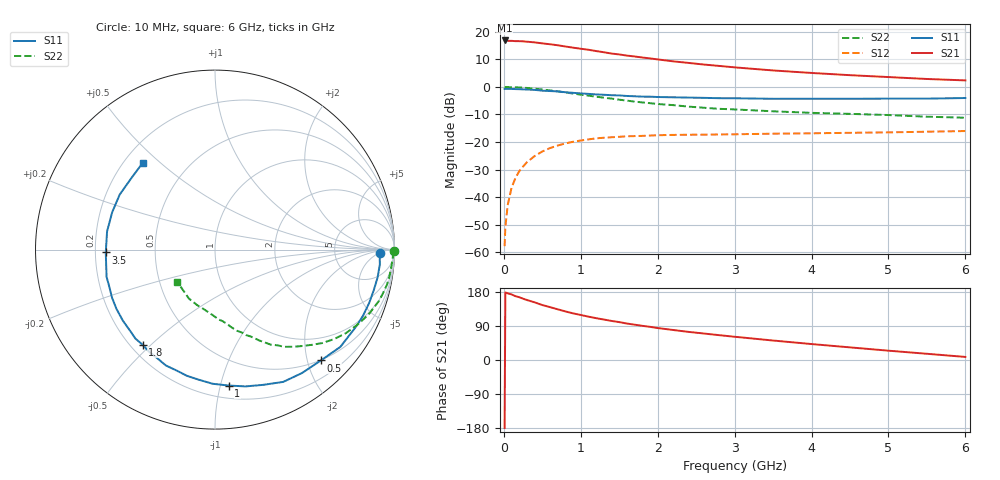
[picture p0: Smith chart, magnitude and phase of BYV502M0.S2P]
! SIEMENS Small Signal Semiconductors
! BFY420
! Si NPN RF SIEGET Grounded Emitter Transistor in MICRO-X
! VCE = 0.5 V  IC = 2 mA
! Common Emitter S-Parameters:  October  1996
# GHz  S  MA  R  50
!  f  S11  S21  S12  S22
! GHz  MAG  ANG  MAG  ANG  MAG  ANG  MAG  ANG
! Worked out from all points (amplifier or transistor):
!   36 points, 10 MHz to 6 GHz, reference 50 ohm
!   highest |S21| = 16.8 dB at 10 MHz (marker M1)
!   |S21| within 3 dB of that: start of sweep to 999.7 MHz
!   unconditionally stable (mu >= 1): 3.915 GHz to end of sweep
!   at 250 MHz: K = 0.06, MSG = 22.7 dB, |S12| = -28.8 dB
!   at 1.4 GHz: K = 0.34, MSG = 15.2 dB, |S12| = -18.3 dB
!   at 6 GHz: K = 1.28, MAG = 6.0 dB, |S12| = -16.0 dB
!   S11 on the Smith chart (normalised r, x): 10 MHz: 22, -5; 500 MHz: 0.49, -2.25; 1 GHz: 0.29, -1.06; 1.8 GHz: 0.25, -0.47; 3.5 GHz: 0.24, -0.01; 6 GHz: 0.27, +0.44
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0.01  0.918 -1.2  6.945 -179.6  0.0013 107.8  0.9948 -0.6
0.02  0.9182 -2.2  6.909 178.3  0.0029 90.0  0.9929 -1.1
0.05  0.9222 -5.1  6.82 175.9  0.0072 84.8  0.9911 -2.9
0.1  0.919 -9.7  6.835 173.1  0.0149 84.5  0.9864 -5.9
0.15  0.913 -14.4  6.75 168.5  0.0222 80.2  0.983 -8.9
0.2  0.909 -19.1  6.743 165.7  0.0297 78.6  0.9778 -11.6
0.3  0.8955 -28.6  6.595 158.3  0.0432 72.7  0.9578 -17.3
0.4  0.884 -37.8  6.413 152.2  0.0558 66.8  0.9294 -22.8
0.5  0.8543 -46.3  6.144 145.0  0.0676 62.3  0.8983 -27.7
0.7  0.8294 -62.7  5.687 133.8  0.0865 52.9  0.83 -36.9
0.9  0.781 -77.4  5.144 123.1  0.1013 44.9  0.7579 -44.4
1  0.7614 -84.2  4.916 118.8  0.1068 41.6  0.7241 -47.9
1.1  0.7476 -91.0  4.713 114.4  0.1119 38.3  0.6938 -51.3
1.4  0.7068 -107.7  4.02 103.1  0.1223 30.1  0.6142 -59.6
1.6  0.6847 -118.3  3.691 96.2  0.1275 26.3  0.5645 -63.9
1.8  0.6658 -127.3  3.408 90.2  0.1297 23.0  0.5239 -67.6
2.2  0.6482 -142.4  2.907 79.2  0.135 16.8  0.4676 -75.0
2.8  0.6242 -160.6  2.399 65.5  0.1376 11.4  0.4007 -84.0
3.5  0.6088 -178.5  1.987 51.4  0.1421 7.1  0.3614 -93.0
4.5  0.6095 160.0  1.631 33.3  0.1473 2.0  0.3248 -107.9
5.5  0.6132 139.3  1.392 16.4  0.1542 -1.7  0.2884 -127.8
6  0.6291 129.8  1.312 8.1  0.1585 -3.1  0.2762 -139.6
